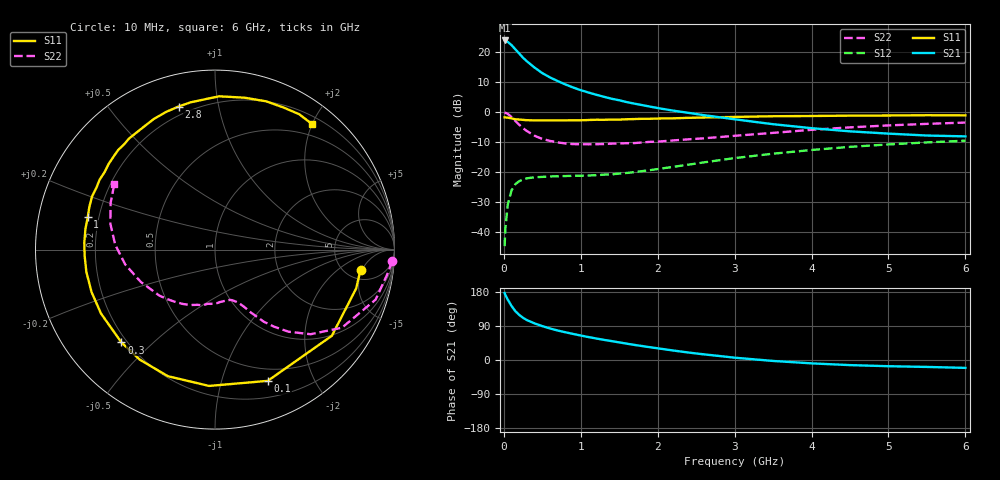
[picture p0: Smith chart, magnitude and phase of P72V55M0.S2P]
! SIEMENS Small Signal Semiconductors
! BFP196
! Si NPN RF Bipolar Junction Transistor in SOT143
! VCE = 2.5 V  IC = 5 mA
! Common Emitter S-Parameters:  May  1996
# GHz  S  MA  R  50
!  f  S11  S21  S12  S22
! GHz  MAG  ANG  MAG  ANG  MAG  ANG  MAG  ANG
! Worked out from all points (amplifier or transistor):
!   36 points, 10 MHz to 6 GHz, reference 50 ohm
!   highest |S21| = 23.9 dB at 10 MHz (marker M1)
!   |S21| within 3 dB of that: start of sweep to 150.7 MHz
!   unconditionally stable (mu >= 1): 1.117 GHz to 3.246 GHz; 5.996847 GHz to end of sweep
!   at 250 MHz: K = 0.25, MSG = 20.3 dB, |S12| = -22.4 dB
!   at 1.4 GHz: K = 1.16, MAG = 10.2 dB, |S12| = -20.8 dB
!   at 6 GHz: K = 1.00, MAG = 0.6 dB, |S12| = -9.5 dB
!   S11 on the Smith chart (normalised r, x): 10 MHz: 6.87, -4.63; 100 MHz: 0.37, -1.42; 300 MHz: 0.18, -0.40; 1 GHz: 0.16, +0.12; 2.8 GHz: 0.16, +0.77; 6 GHz: 0.31, +2.00
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0.01  0.8187 -7.8  15.71 176.8  0.0058 86.8  0.9878 -3.7
0.02  0.8157 -15.4  15.47 171.4  0.0114 81.6  0.9753 -7.1
0.05  0.809 -36.4  14.9 159.7  0.0282 71.9  0.9373 -17.3
0.1  0.7881 -68.1  13.15 142.6  0.0496 56.9  0.8304 -31.6
0.15  0.7603 -92.5  11.15 128.7  0.0628 45.9  0.7114 -41.5
0.2  0.7525 -110.4  9.512 119.0  0.0705 38.5  0.6148 -48.1
0.25  0.7428 -124.4  8.077 111.2  0.0755 32.8  0.5388 -52.7
0.3  0.7344 -135.2  7.042 105.3  0.0787 29.7  0.4833 -56.0
0.4  0.7282 -150.7  5.533 96.5  0.0817 24.9  0.4033 -60.3
0.5  0.7274 -161.0  4.48 89.4  0.0831 22.5  0.3572 -63.1
0.6  0.7274 -170.1  3.798 83.2  0.0845 21.3  0.3312 -65.4
0.7  0.7273 -177.4  3.298 77.8  0.0851 20.9  0.3128 -68.0
0.8  0.7293 176.8  2.899 73.2  0.0858 21.1  0.3005 -70.6
1  0.7315 165.7  2.325 64.6  0.0866 22.9  0.2909 -75.7
1.1  0.7393 161.3  2.125 60.5  0.0877 24.1  0.2908 -78.7
1.6  0.7608 141.2  1.469 43.0  0.0967 31.8  0.3032 -94.3
2.2  0.7881 121.7  1.061 25.1  0.122 38.7  0.337 -113.7
2.8  0.8227 104.3  0.823 10.6  0.1576 39.2  0.3835 -134.0
3.5  0.8544 88.5  0.629 -2.5  0.2026 33.9  0.451 -156.5
4.5  0.8741 70.9  0.478 -13.5  0.2637 22.6  0.5571 177.1
5.5  0.8883 58.1  0.407 -18.3  0.3126 10.1  0.6372 155.9
6  0.8839 52.3  0.394 -20.8  0.3337 3.4  0.6701 146.8
